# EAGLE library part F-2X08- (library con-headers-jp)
FEMALE HEADER
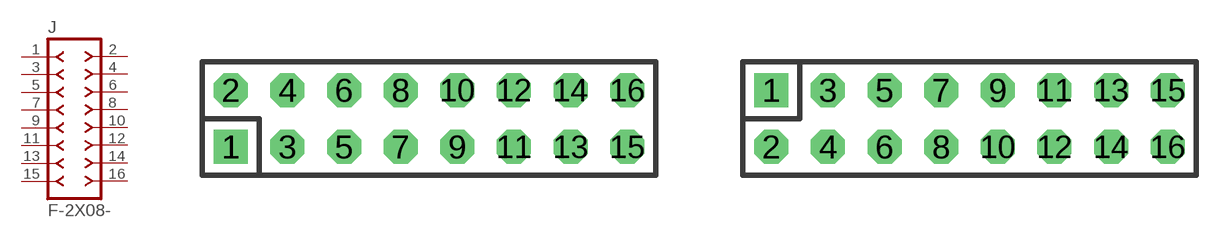
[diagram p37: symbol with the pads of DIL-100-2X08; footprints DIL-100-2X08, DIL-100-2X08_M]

Designator prefix J

## F-2X08-DIL-100  [DIL-100-2X08]
1  1  pas
2  2  pas
3  3  pas
4  4  pas
5  5  pas
6  6  pas
7  7  pas
8  8  pas
9  9  pas
10  10  pas
11  11  pas
12  12  pas
13  13  pas
14  14  pas
15  15  pas
16  16  pas

## F-2X08-DIL-100_M  [DIL-100-2X08_M]
Pads as for DIL-100-2X08

## F-2X08-DIL-2MM  [DIL-2MM-2X08]
Pads as for DIL-100-2X08

## F-2X08-DIL-2MM_M  [DIL-2MM-2X08_M]
Pads as for DIL-100-2X08

## F-2X08-71991  [71991-16]
Pads as for DIL-100-2X08

## F-2X08-79107  [79107-16]
Pads as for DIL-100-2X08

## F-2X08-79107_M  [79107-16_M]
Pads as for DIL-100-2X08

## Footprint DIL-100-2X08 (pad centres in mm)
PIN HEADER - 0.1"
drill 1.016 square: 1 -8.89,-1.27
drill 1.016 octagon: 2 -8.89,1.27; 3 -6.35,-1.27; 4 -6.35,1.27; 5 -3.81,-1.27; 6 -3.81,1.27; 7 -1.27,-1.27; 8 -1.27,1.27; 9 1.27,-1.27; 10 1.27,1.27; 11 3.81,-1.27; 12 3.81,1.27; 13 6.35,-1.27; 14 6.35,1.27; 15 8.89,-1.27; 16 8.89,1.27

## Footprint DIL-100-2X08_M (pad centres in mm)
PIN HEADER - MIRRORED 0.1"
drill 1.016 square: 1 -8.89,1.27
drill 1.016 octagon: 2 -8.89,-1.27; 3 -6.35,1.27; 4 -6.35,-1.27; 5 -3.81,1.27; 6 -3.81,-1.27; 7 -1.27,1.27; 8 -1.27,-1.27; 9 1.27,1.27; 10 1.27,-1.27; 11 3.81,1.27; 12 3.81,-1.27; 13 6.35,1.27; 14 6.35,-1.27; 15 8.89,1.27; 16 8.89,-1.27

## Footprint DIL-2MM-2X08 (pad centres in mm)
PIN HEADER - 2MM"
drill 0.711 square: 1 -7,-1
drill 0.711: 2 -7,1; 3 -5,-1; 4 -5,1; 5 -3,-1; 6 -3,1; 7 -1,-1; 8 -1,1; 9 1,-1; 10 1,1; 11 3,-1; 12 3,1; 13 5,-1; 14 5,1; 15 7,-1; 16 7,1

## Footprint DIL-2MM-2X08_M (pad centres in mm)
PIN HEADER - MIRRORED 2MM
drill 0.711 square: 1 -7,1
drill 0.711: 2 -7,-1; 3 -5,1; 4 -5,-1; 5 -3,1; 6 -3,-1; 7 -1,1; 8 -1,-1; 9 1,1; 10 1,-1; 11 3,1; 12 3,-1; 13 5,1; 14 5,-1; 15 7,1; 16 7,-1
